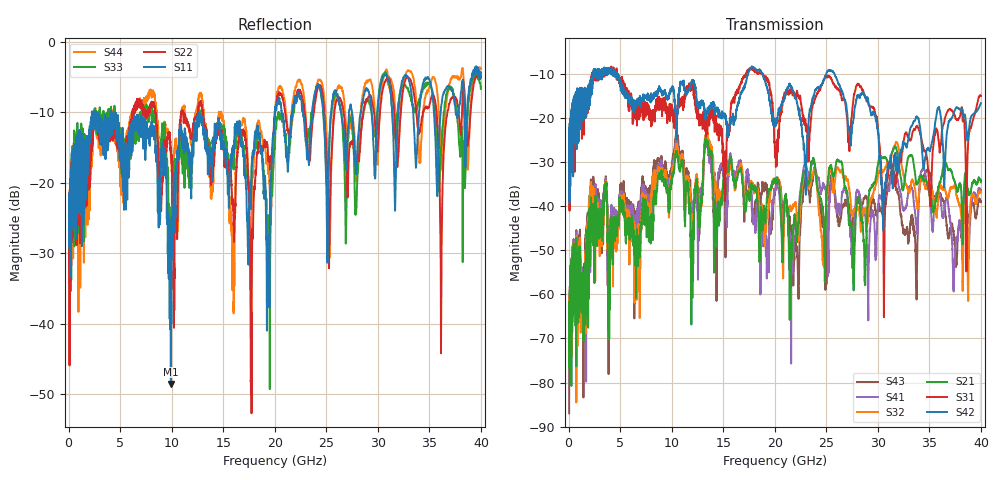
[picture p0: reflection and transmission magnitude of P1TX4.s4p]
!Agilent Technologies,N5245A,MY49151084,A.09.20.08
!Agilent N5245A: A.09.20.08
!Date: Thursday, March 01, 2012 11:55:33
!Correction: S11(Full 4 Port(1,2,3,4))
!S12(Full 4 Port(1,2,3,4))
!S13(Full 4 Port(1,2,3,4))
!S14(Full 4 Port(1,2,3,4))
!S21(Full 4 Port(1,2,3,4))
!S22(Full 4 Port(1,2,3,4))
!S23(Full 4 Port(1,2,3,4))
!S24(Full 4 Port(1,2,3,4))
!S31(Full 4 Port(1,2,3,4))
!S32(Full 4 Port(1,2,3,4))
!S33(Full 4 Port(1,2,3,4))
!S34(Full 4 Port(1,2,3,4))
!S41(Full 4 Port(1,2,3,4))
!S42(Full 4 Port(1,2,3,4))
!S43(Full 4 Port(1,2,3,4))
!S44(Full 4 Port(1,2,3,4))
!S4P File: Measurements: <S11,S12,S13,S14>,
!<S21,S22,S23,S24>,
!<S31,S32,S33,S34>,
!<S41,S42,S43,S44>:
# Hz S  dB  R 50
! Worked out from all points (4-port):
!   3996 points, 50 MHz to 40 GHz, reference 50 ohm
!   strongest paths, dB at 50 MHz, 10.04 GHz, 20.03 GHz, 30.02 GHz, 40 GHz:
!     S42: -27.1, -13.4, -21.7, -23.6, -16.7
!     S31: -26.4, -18.6, -28.0, -22.5, -15.0
!     S21: -63.8, -34.0, -34.4, -30.6, -34.6
!     S32: -76.7, -32.5, -34.1, -32.8, -36.9
!     S41: -63.1, -31.8, -36.2, -40.4, -36.7
!     S43: -87.0, -30.1, -36.8, -40.1, -39.2
!   lowest |S11| = -48.5 dB at 9.92 GHz (marker M1), VSWR 1.01, Z = 49.6 + j0.084 ohm
!   |S11| at or under -10 dB: start of sweep to 2.258 GHz; 2.64 GHz to 4.09 GHz (1.45 GHz wide, 43.1 % of centre); 4.33 GHz to 20.03 GHz (15.7 GHz wide, 129 % of centre)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
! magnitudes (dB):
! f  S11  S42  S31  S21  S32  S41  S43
! 50 MHz  -25.1  -27.1  -26.4  -63.8  -76.7  -63.1  -87.0
! 2.28 GHz  -10.1  -12.7  -11.1  -42.3  -37.0  -42.2  -36.1
! 9.92 GHz  -48.5  -13.7  -18.1  -35.4  -34.2  -33.9  -32.1
! 28.18 GHz  -12.2  -15.1  -12.4  -38.4  -40.8  -37.5  -39.1
! 30.62 GHz  -4.8  -37.0  -54.7  -29.0  -31.8  -38.8  -41.7
! 36.15 GHz  -9.1  -20.4  -25.0  -33.6  -35.8  -39.6  -38.2
! 40 GHz  -5.1  -16.7  -15.0  -34.6  -36.9  -36.7  -39.2
